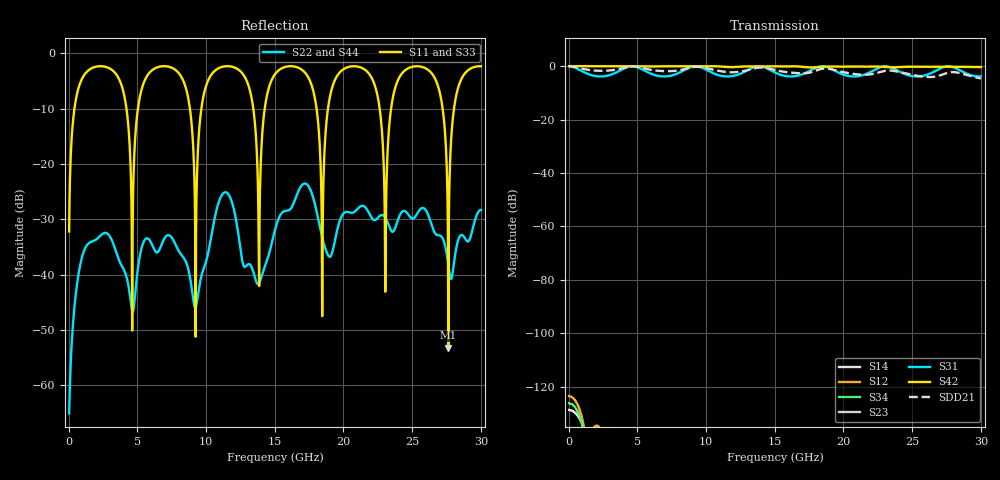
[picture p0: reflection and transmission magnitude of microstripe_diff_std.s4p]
! TOUCHSTONE file generated by CST MICROWAVE STUDIO
! Date and time: Tue Jan 25 17:16:37 2011
! Project name: microstripe_diff_std.cst
# GHZ S MA R 50
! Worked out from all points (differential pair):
!   1000 points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, 30 MHz to 30 GHz, reference 50 ohm
!   strongest paths, dB at 30 MHz, 7.53 GHz, 15.03 GHz, 22.53 GHz, 30 GHz:
!     S42: 0.0, -0.1, -0.1, -0.1, -0.3
!     S31: 0.0, -3.4, -2.4, -0.7, -3.8
!     S23: -146.0, -149.1, -148.5, -146.4, -152.3
!     S34: -126.2, -148.8, -154.9, -139.2, -143.8
!     S12: -123.6, -147.9, -148.8, -143.1, -139.5
!     S14: -128.8, -152.9, -148.2, -145.9, -137.0
!   taken as a pair (ports 2,1 in; 4,3 out), SDD21 dB: 0.0, -1.8, -1.5, -2.4, -4.6
!   lowest |S11| = -53.2 dB at 27.63 GHz (marker M1), VSWR 1.00, Z = 50.2 + j0.0365 ohm
!   |S11| at or under -10 dB: 8.823 GHz to 9.654 GHz (830.8 MHz wide, 8.99 % of centre); 13.44 GHz to 14.27 GHz (829.6 MHz wide, 5.99 % of centre); 22.63 GHz to 23.46 GHz (827.4 MHz wide, 3.59 % of centre)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
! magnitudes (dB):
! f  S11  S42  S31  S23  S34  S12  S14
! 30 MHz  -32.2  0.0  0.0  -146.0  -126.2  -123.6  -128.8
! 2.55 GHz  -2.3  0.0  -3.8  -149.5  -143.5  -140.3  -140.9
! 9.24 GHz  -51.2  -0.1  0.0  -146.3  -149.2  -162.4  -157.8
! 10.86 GHz  -2.7  -0.1  -3.3  -150.1  -151.7  -165.6  -156.3
! 25.86 GHz  -2.6  -0.2  -3.5  -147.0  -143.7  -149.6  -145.7
! 27.63 GHz  -53.2  -0.3  0.0  -143.0  -139.3  -145.4  -141.9
! 30 GHz  -2.3  -0.3  -3.8  -152.3  -143.8  -139.5  -137.0
